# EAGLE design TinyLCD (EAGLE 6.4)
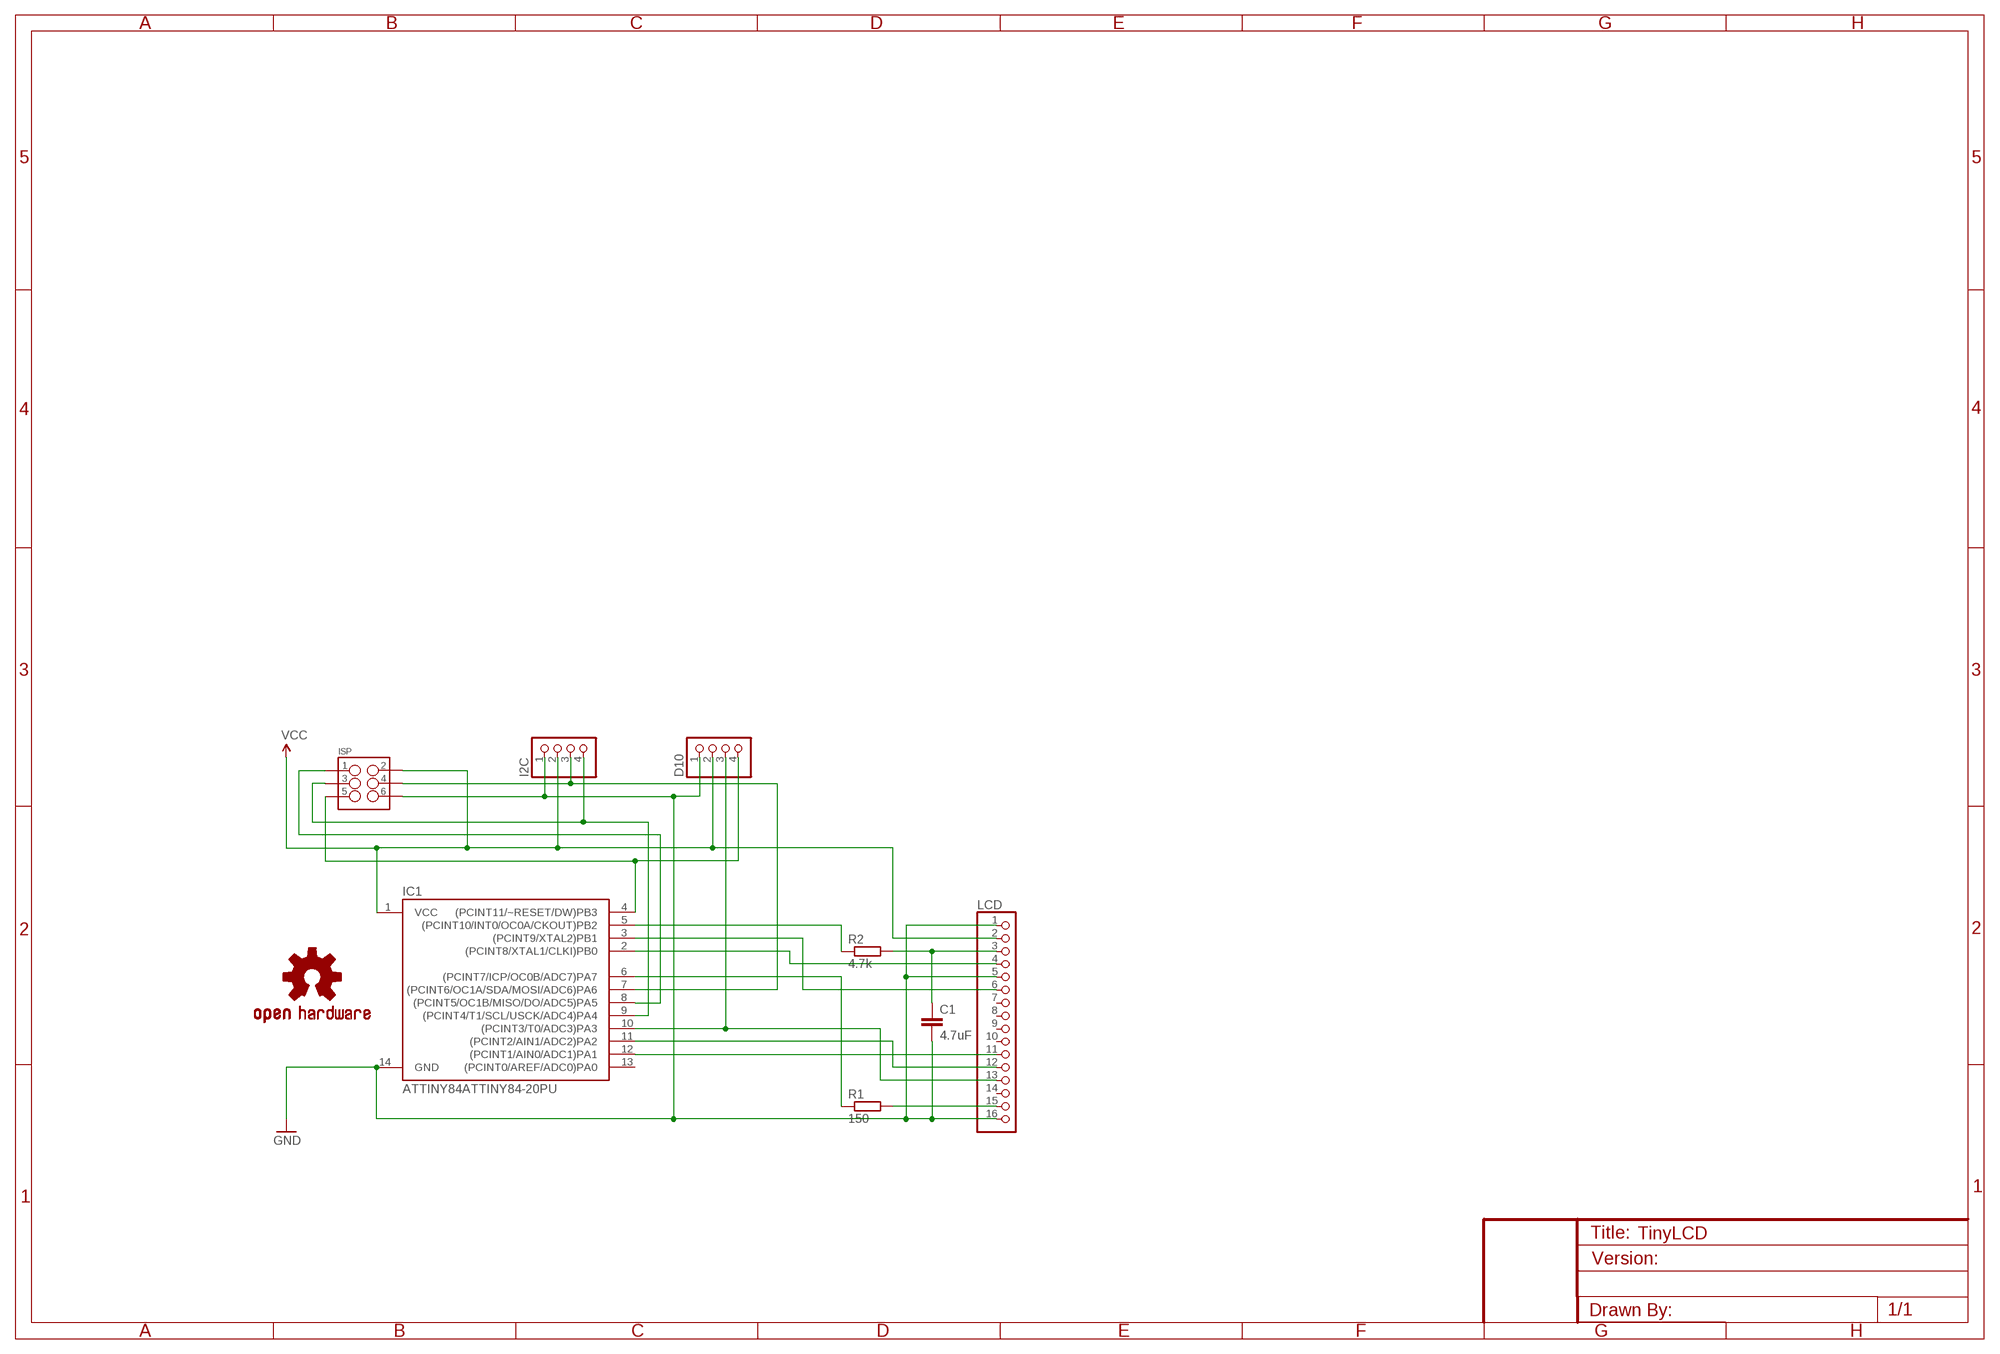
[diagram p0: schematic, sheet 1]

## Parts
C1  4.7uF  C-EU025-030X050  [C025-030X050]
D10  PINHD-1X4  [1X04]
I2C  PINHD-1X4  [1X04]
IC1  ATTINY84ATTINY84-20PU  [DIL14]
ISP  M03X2  [2X3-SHROUDED]
LCD  PINHD-1X16  [1X16]
LOGO1  OSHW-LOGOS  [OSHW-LOGO-S]
R1  150  R-EU_0207/10  [0207/10]
R2  4.7k  R-EU_0207/10  [0207/10]

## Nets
GND: C1.2 D10.1 I2C.1 IC1.14(GND) ISP.6 LCD.1 LCD.5 LCD.16
N$1: IC1.2((PCINT8/XTAL1/CLKI)PB0) LCD.4
N$2: IC1.3((PCINT9/XTAL2)PB1) LCD.6
N$3: C1.1 LCD.3 R2.2
N$4: IC1.5((PCINT10/INT0/OC0A/CKOUT)PB2) R2.1
N$5: D10.4 IC1.4((PCINT11/~RESET/DW)PB3) ISP.5
N$6: I2C.3 IC1.7((PCINT6/OC1A/SDA/MOSI/ADC6)PA6) ISP.4
N$8: LCD.15 R1.2
N$9: IC1.6((PCINT7/ICP/OC0B/ADC7)PA7) R1.1
N$10: I2C.4 IC1.9((PCINT4/T1/SCL/USCK/ADC4)PA4) ISP.3
N$11: IC1.8((PCINT5/OC1B/MISO/DO/ADC5)PA5) ISP.1
N$12: IC1.11((PCINT2/AIN1/ADC2)PA2) LCD.12
N$13: IC1.12((PCINT1/AIN0/ADC1)PA1) LCD.11
N$14: D10.3 IC1.10((PCINT3/T0/ADC3)PA3) LCD.13
VCC: D10.2 I2C.2 IC1.1(VCC) ISP.2 LCD.2
Unconnected: IC1.13((PCINT0/AREF/ADC0)PA0) LCD.7 LCD.8 LCD.9 LCD.10 LCD.14

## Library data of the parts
C1 = rcl:C-EU: CAPACITOR, European symbol
D10 I2C = pinhead:PINHD-1X4: PIN HEADER
IC1 = SparkFun-DigitalIC:ATTINY84: Atmel 14-pin 2/4/8kB flash uC
ISP = SparkFun-Connectors:M03X2: 2x3 .1" header. Shrouded, with keying- CONN-10681 SMT- CONN-11415 Pogo pins- HW-11044; PROD_ID: CONN-10681
LCD = pinhead:PINHD-1X16: PIN HEADER
LOGO1 = SparkFun-Aesthetics:OSHW-LOGO: Open Source Hardware Logo This logo indicates the piece of hardware it is found on incorporates a OSHW license and/or adheres to the definition of open source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
R1 R2 = rcl:R-EU_: RESISTOR, European symbol

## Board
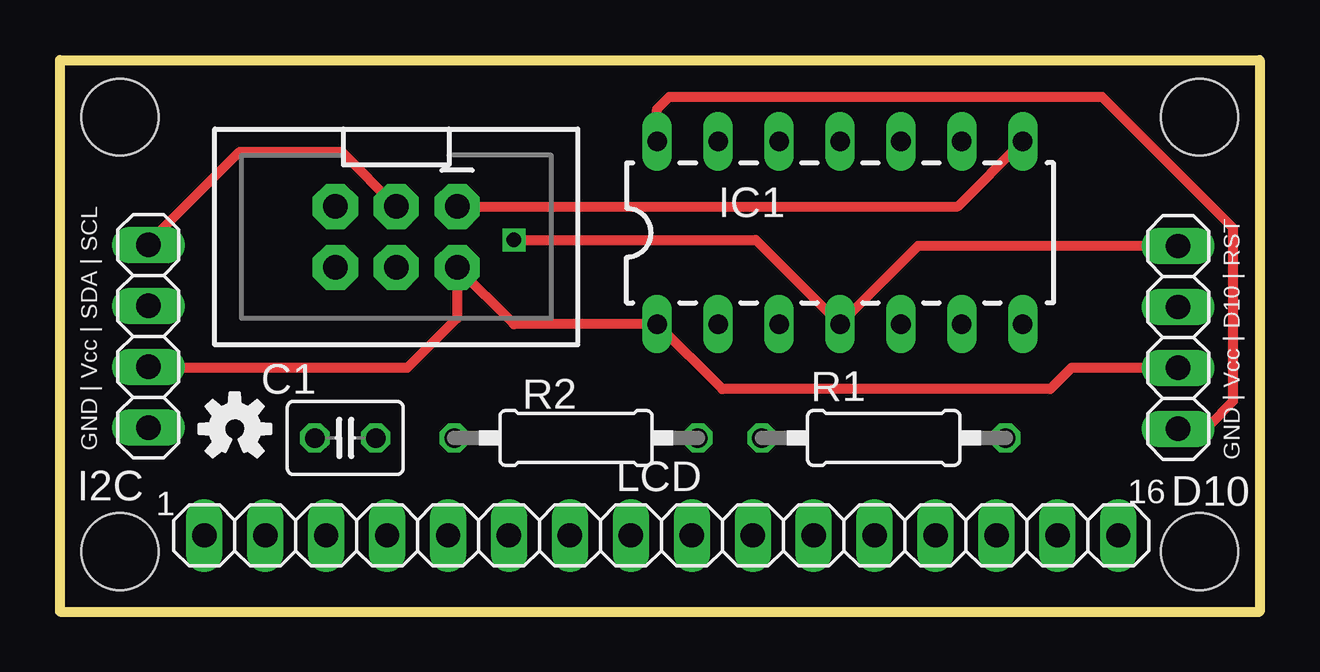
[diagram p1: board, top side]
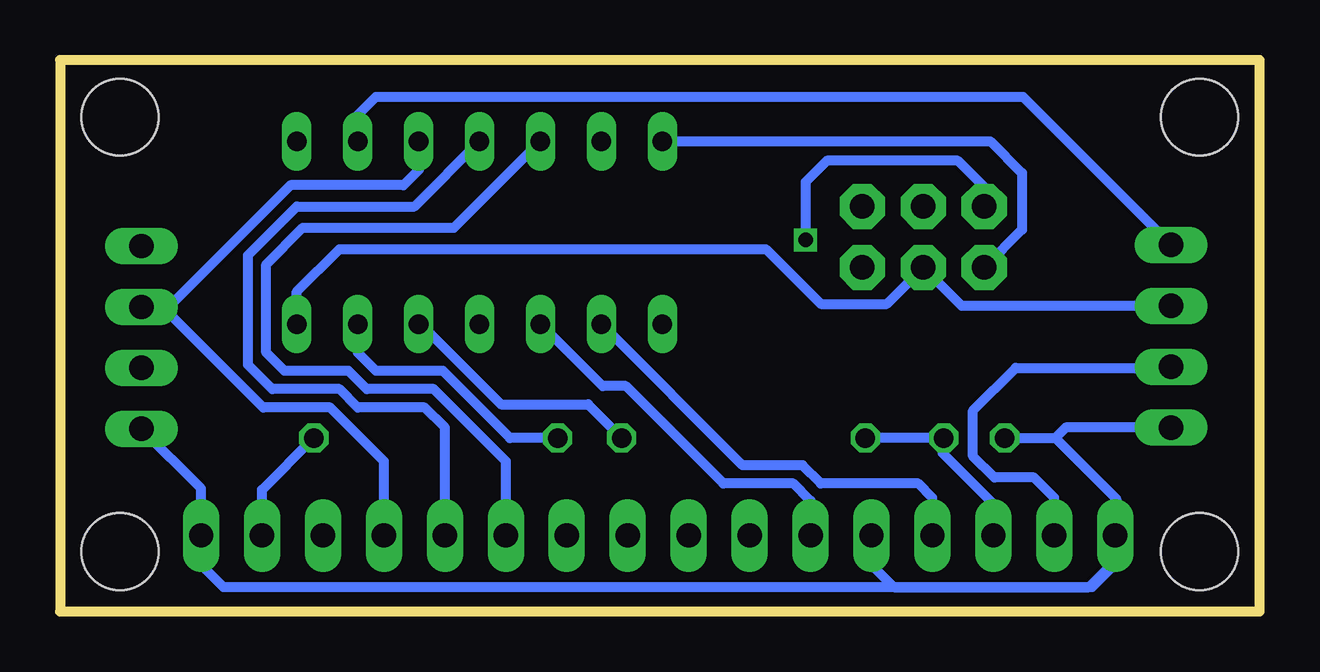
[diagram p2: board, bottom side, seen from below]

Size 50 x 23 mm. Coordinates in mm from the lower left corner, seen from the top.
Outline: 0,0 50,0 50,23 0,23 0,0
Copper layers (1*16): Top 0.0356mm / dielectric 1.5011mm / Bottom 0.0356mm
Design rules "LaenPCBOrder": minimum track width 6mil, minimum drill 13mil, track to track 6mil, track to pad 6mil, pad to pad 6mil, via to via 6mil, smd to smd 6mil, copper to edge 15mil, drill to drill 6mil, minimum pad ring 7mil, minimum via ring 7mil, stop-mask expansion 4mil, vias tented up to drill 0mil, thermal gap 10mil
Holes 3.2 mm at 2.5,2.5 47.5,2.5 47.5,20.62 2.5,20.62

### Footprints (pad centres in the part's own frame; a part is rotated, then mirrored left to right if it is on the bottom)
C025-030X050 = drill 0.813 octagon: 1 -1.27,0; 2 1.27,0
1X04 = drill 1.016 long: 1 -3.81,0; 2 -1.27,0; 3 1.27,0; 4 3.81,0
DIL14 = drill 0.813 long: 1 -8.89,-3.81; 2 -6.35,-3.81; 3 -3.81,-3.81; 4 -1.27,-3.81; 5 1.27,-3.81; 6 3.81,-3.81; 7 6.35,-3.81; 8 6.35,3.81; 9 3.81,3.81; 10 1.27,3.81; 11 -1.27,3.81; 12 -3.81,3.81; 13 -6.35,3.81; 14 -8.89,3.81
2X3-SHROUDED = drill 1.016 pad 1.88 octagon: 1 -1.27,2.54; 2 1.27,2.54; 3 -1.27,0; 4 1.27,0; 5 -1.27,-2.54; 6 1.27,-2.54
1X16 = drill 1.016 long: 1 -19.05,0; 2 -16.51,0; 3 -13.97,0; 4 -11.43,0; 5 -8.89,0; 6 -6.35,0; 7 -3.81,0; 8 -1.27,0; 9 1.27,0; 10 3.81,0; 11 6.35,0; 12 8.89,0; 13 11.43,0; 14 13.97,0; 15 16.51,0; 16 19.05,0
0207/10 = drill 0.813 octagon: 1 -5.08,0; 2 5.08,0

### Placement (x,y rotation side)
C1  11.89,7.24 180 top
D10  46.61,11.43 90 top
I2C  3.68,11.48 90 top
IC1  33.78,15.79 0 top
ISP  14.02,15.62 270 top
LCD  25.07,3.17 0 top
LOGO1  7.29,7.62 0 top
R1  34.34,7.24 0 top
R2  21.51,7.24 180 top

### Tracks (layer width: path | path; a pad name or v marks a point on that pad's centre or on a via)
GND
  Top 0.406: IC1.14 24.89,20.95 25.4,21.46 43.43,21.46 48.9,16 48.9,8.76 47.88,7.75 46.74,7.75 D10.1
  Bottom 0.406: D10.1 44.12,5.13 LCD.16 44.2,3.1 44.2,2.03 43.18,1.02 6.99,1.02 5.97,2.03 5.97,2.16 | 6.02,4.75 LCD.1 5.97,3.13 | 6.02,4.75 8.51,7.24 | I2C.1 8.08,7.67 8.51,7.24 | IC1.14 11.22,19.61 9.91,18.29 9.91,15.92 ISP.6 | LCD.5 16.18,1.95 15.24,1.02 7.11,1.02 5.97,2.16 | 5.97,2.16 5.97,3.13 | C1.2 8.51,7.24 | 6.02,4.75 5.97,4.7 5.97,3.13
N$1
  Bottom 0.406: LCD.4 13.64,4.75 14.22,5.33 18.29,5.33 19.05,6.1 21.54,6.1 IC1.2
N$2
  Bottom 0.406: LCD.6 18.72,4.62 19.43,5.33 22.35,5.33 26.42,9.4 27.39,9.4 IC1.3
N$3
  Bottom 0.406: LCD.3 11.1,4.49 13.21,6.6 13.21,7.19 C1.1 R2.2
N$4
  Bottom 0.406: IC1.5 34.97,11.98 31.62,8.64 27.99,8.64 R2.1
N$5  (via drill 0.6)
  Top 0.406: v18.92,15.49 29,15.49 IC1.4 35.77,15.24 D10.4
  Bottom 0.406: ISP.5 11.48,17.7 12.57,18.8 18.03,18.8 18.92,17.91 v18.92,15.49
N$6
  Bottom 0.406: IC1.7 40.13,13.34 38.35,15.11 20.57,15.11 18.29,12.83 15.54,12.83 ISP.4 12.41,12.75 I2C.3
N$8
  Bottom 0.406: LCD.15 41.58,5.08 R1.2
N$9
  Bottom 0.406: IC1.6 37.59,10.79 36.83,10.03 34.04,10.03 31.24,7.24 R1.1
N$10
  Top 0.406: I2C.4 3.68,15.37 7.49,19.18 11.73,19.18 ISP.3
  Bottom 0.406: IC1.9 37.59,20.7 36.83,21.46 9.86,21.46 I2C.4
N$11
  Top 0.406: ISP.1 37.42,16.89 IC1.8
N$12
  Bottom 0.406: LCD.12 33.96,7.67 34.8,8.51 37.59,8.51 38.35,9.27 41.15,9.27 42.16,10.29 42.16,14.86 40.13,16.89 35.23,16.89 IC1.11
N$13
  Bottom 0.406: IC1.12 33.58,16 39.88,16 41.4,14.48 41.4,10.79 40.64,10.03 37.97,10.03 37.21,9.27 34.42,9.27 31.42,6.27 LCD.11
N$14
  Bottom 0.406: LCD.13 36.5,6.27 38.73,8.51 41.53,8.51 45.59,12.57 | 45.59,12.57 46.48,12.57 D10.3 | IC1.10 35.05,18.41 35.69,17.78 40.39,17.78 45.59,12.57
VCC
  Top 0.406: I2C.2 3.73,10.16 14.48,10.16 16.56,12.24 ISP.2 18.92,11.98 IC1.1 27.61,9.27 41.27,9.27 42.16,10.16 D10.2
  Bottom 0.406: LCD.2 8.56,4.75 9.4,5.59 11.05,5.59 11.94,6.48 11.94,8.38 10.16,10.16 3.73,10.16 I2C.2

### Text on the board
tNames: GND | Vcc | SDA | SCL | GND | Vcc | D10 | RST | 1 | 16

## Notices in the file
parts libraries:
SparkFun-Aesthetics: Licensing: CC v3.0 Share-Alike You are welcome to use this library for commercial purposes.
